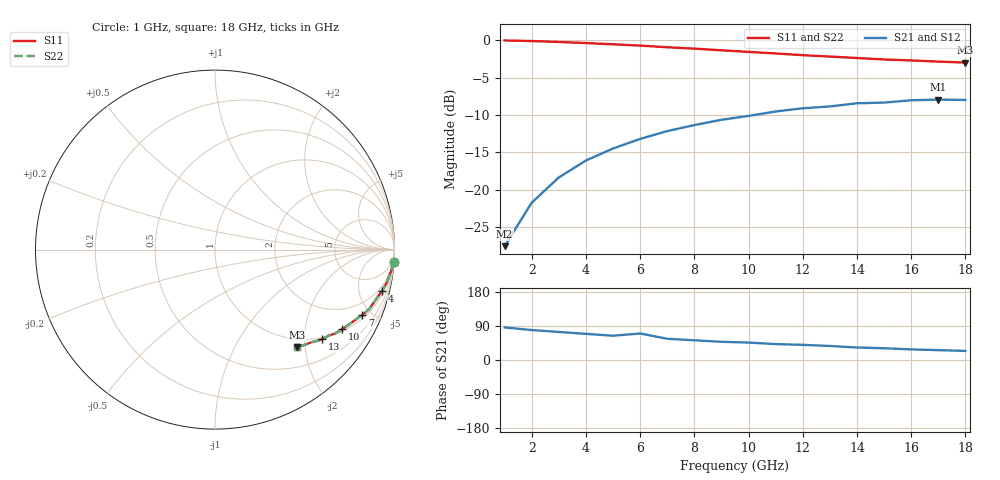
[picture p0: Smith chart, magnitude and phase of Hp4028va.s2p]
!HPND-4028 beam lead PIN diode
!Series configuration S-parameters Vr= 0 V.  Last updated 10/3/97
# mhz s ma r 50
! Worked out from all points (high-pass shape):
!   18 points, 1 GHz to 18 GHz, reference 50 ohm
!   highest |S21| = -7.94 dB at 17 GHz (marker M1); lowest = -27.5 dB at 1 GHz (marker M2)
!   |S21| within 3 dB of the highest: 8.57 GHz to end of sweep
!   lowest |S11| = -3.0 dB at 18 GHz (marker M3), VSWR 5.87, Z = 42.1 - j91.9 ohm
!   |S11| at or under -10 dB: nowhere
!   |S22| runs from -3.0 to 0.0 dB; largest |S21 - S12| = 0
!   S11 on the Smith chart (normalised r, x): 1 GHz: 1, -29; 4 GHz: 1.40, -7.90; 7 GHz: 1.17, -4.41; 10 GHz: 1.07, -3.15; 13 GHz: 0.95, -2.42; 18 GHz: 0.84, -1.84
1000  0.997 -4.0  0.042 86.0  0.042 86.0  0.997 -4.0
2000  0.988 -7.0  0.082 79.0  0.082 79.0  0.988 -7.0
3000  0.974 -11.0  0.121 74.0  0.121 74.0  0.974 -11.0
4000  0.958 -14.0  0.157 69.0  0.157 69.0  0.958 -14.0
5000  0.94 -17.0  0.189 64.0  0.189 64.0  0.94 -17.0
6000  0.921 -21.0  0.219 70.0  0.219 70.0  0.921 -21.0
7000  0.898 -24.0  0.247 56.0  0.247 56.0  0.898 -24.0
8000  0.879 -26.0  0.271 52.0  0.271 52.0  0.879 -26.0
9000  0.857 -29.0  0.294 48.0  0.294 48.0  0.857 -29.0
10000  0.836 -32.0  0.312 46.0  0.312 46.0  0.836 -32.0
11000  0.816 -35.0  0.334 42.0  0.334 42.0  0.816 -35.0
12000  0.795 -37.0  0.351 40.0  0.351 40.0  0.795 -37.0
13000  0.778 -40.0  0.361 37.0  0.361 37.0  0.778 -40.0
14000  0.761 -42.0  0.379 33.0  0.379 33.0  0.761 -42.0
15000  0.744 -44.0  0.383 31.0  0.383 31.0  0.744 -44.0
16000  0.733 -46.0  0.397 28.0  0.397 28.0  0.733 -46.0
17000  0.72 -48.0  0.401 26.0  0.401 26.0  0.72 -48.0
18000  0.709 -50.0  0.399 24.0  0.399 24.0  0.709 -50.0
